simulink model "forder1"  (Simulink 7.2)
settings: Solver=ode45  StartTime=0.0  StopTime=10.0  RelTol=1e-3
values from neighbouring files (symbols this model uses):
  k = 1    [second_init.m]
  ki = 1    [second_init.m]
  tau = 1    [second_init.m]
libraries: simulink x1

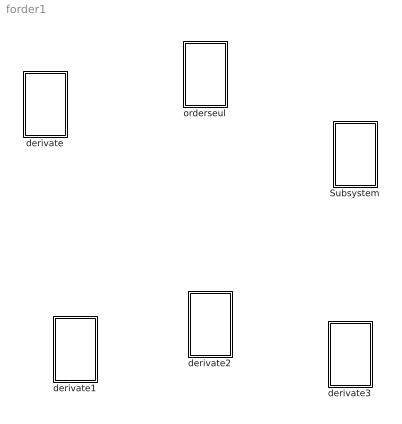
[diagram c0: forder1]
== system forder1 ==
  Subsystem : Subsystem
  derivate : Subsystem
  derivate1 : Subsystem
  derivate2 : Subsystem
  derivate3 : Subsystem
  orderseul : Subsystem

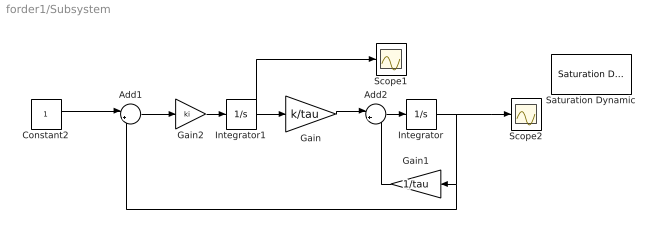
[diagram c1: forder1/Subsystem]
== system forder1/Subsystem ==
  Add1 : Sum  Inputs=|+-  OutDataType=sfix(16)  OutScaling=2^-10
  Add2 : Sum  Inputs=|+-  OutDataType=sfix(16)  OutScaling=2^-10
  Constant2 : Constant  OutDataType=sfix(16)  OutScaling=2^0
  Gain : Gain  Gain=k/tau  ParameterDataType=sfix(16)  ParameterScaling=2^0  OutDataType=sfix(16)  OutScaling=2^0
  Gain1 : Gain  Orientation=left  Gain=1/tau  ParameterDataType=sfix(16)  ParameterScaling=2^0  OutDataType=sfix(16)  OutScaling=2^0
  Gain2 : Gain  Gain=ki  ParameterDataType=sfix(16)  ParameterScaling=2^0  OutDataType=sfix(16)  OutScaling=2^0
  Integrator : Integrator
  Integrator1 : Integrator
  Saturation Dynamic : simulink/Discontinuities/Saturation Dynamic  SystemSampleTime=-1  OutMin=[]  OutMax=[]  OutDataTypeStr=Inherit: Same as second input  OutDataType=sfix(16)  OutScaling=2^-10  DoSatur=off
  Scope1 : Scope
  Scope2 : Scope
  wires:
  Constant2/1 -> Add1/1
  Integrator/1 -> Scope2/1, Gain1/1, Add1/2
  Gain1/1 -> Add2/2
  Gain/1 -> Add2/1
  Add2/1 -> Integrator/1
  Integrator1/1 -> Gain/1, Scope1/1
  Gain2/1 -> Integrator1/1
  Add1/1 -> Gain2/1

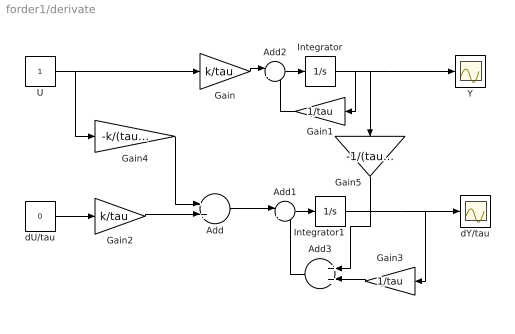
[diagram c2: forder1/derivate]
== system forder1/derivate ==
  Add : Sum  OutDataType=sfix(16)  OutScaling=2^-10
  Add1 : Sum  Inputs=|+-  OutDataType=sfix(16)  OutScaling=2^-10
  Add2 : Sum  Inputs=|+-  OutDataType=sfix(16)  OutScaling=2^-10
  Add3 : Sum  Orientation=left  OutDataType=sfix(16)  OutScaling=2^-10
  Gain : Gain  Gain=k/tau  ParameterDataType=sfix(16)  ParameterScaling=2^0  OutDataType=sfix(16)  OutScaling=2^0
  Gain1 : Gain  Orientation=left  Gain=1/tau  ParameterDataType=sfix(16)  ParameterScaling=2^0  OutDataType=sfix(16)  OutScaling=2^0
  Gain2 : Gain  Gain=k/tau  ParameterDataType=sfix(16)  ParameterScaling=2^0  OutDataType=sfix(16)  OutScaling=2^0
  Gain3 : Gain  Orientation=left  Gain=1/tau  ParameterDataType=sfix(16)  ParameterScaling=2^0  OutDataType=sfix(16)  OutScaling=2^0
  Gain4 : Gain  Gain=-k/(tau^2)  ParameterDataType=sfix(16)  ParameterScaling=2^0  OutDataType=sfix(16)  OutScaling=2^0
  Gain5 : Gain  Orientation=down  Gain=-1/(tau^2)  ParameterDataType=sfix(16)  ParameterScaling=2^0  OutDataType=sfix(16)  OutScaling=2^0
  Integrator : Integrator
  Integrator1 : Integrator
  U : Constant  OutDataType=sfix(16)  OutScaling=2^0
  Y : Scope
  dU/tau : Constant  Value=0  OutDataType=sfix(16)  OutScaling=2^0
  dY/tau : Scope
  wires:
  Integrator/1 -> Y/1, Gain1/1, Gain5/1
  Gain1/1 -> Add2/2
  Gain/1 -> Add2/1
  Add2/1 -> Integrator/1
  U/1 -> Gain/1, Gain4/1
  Integrator1/1 -> dY/tau/1, Gain3/1
  Add1/1 -> Integrator1/1
  dU/tau/1 -> Gain2/1
  Gain2/1 -> Add/2
  Gain4/1 -> Add/1
  Gain3/1 -> Add3/2
  Gain5/1 -> Add3/1
  Add3/1 -> Add1/2
  Add/1 -> Add1/1

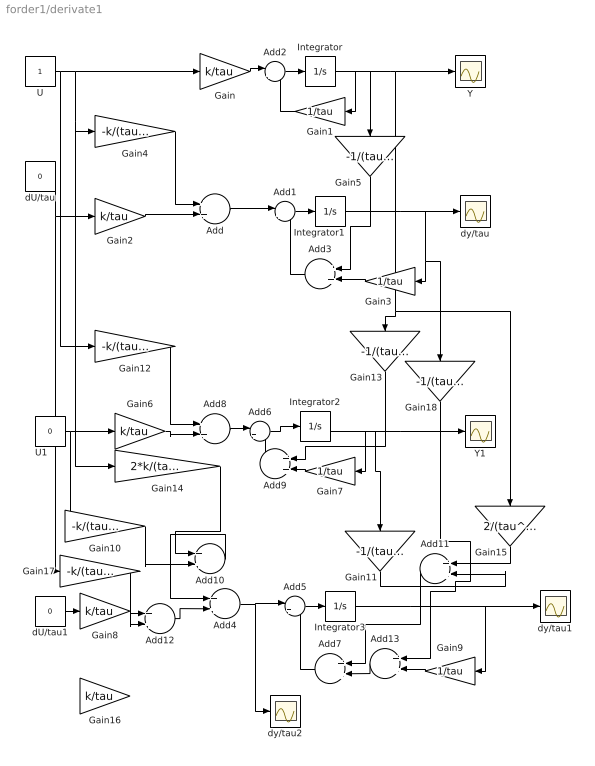
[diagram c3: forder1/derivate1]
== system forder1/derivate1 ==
  Add{,4,8,10,12} (5 alike) : Sum  OutDataType=sfix(16)  OutScaling=2^-10
  Add{1..2,5..6} (4 alike) : Sum  Inputs=|+-  OutDataType=sfix(16)  OutScaling=2^-10
  Add{3,7,9,11,13} (5 alike) : Sum  Orientation=left  OutDataType=sfix(16)  OutScaling=2^-10
  Gain{,2,6,8,16} (5 alike) : Gain  Gain=k/tau  ParameterDataType=sfix(16)  ParameterScaling=2^0  OutDataType=sfix(16)  OutScaling=2^0
  Gain{1,3,7,9} (4 alike) : Gain  Orientation=left  Gain=1/tau  ParameterDataType=sfix(16)  ParameterScaling=2^0  OutDataType=sfix(16)  OutScaling=2^0
  Gain{4,10,12,17} (4 alike) : Gain  Gain=-k/(tau^2)  ParameterDataType=sfix(16)  ParameterScaling=2^0  OutDataType=sfix(16)  OutScaling=2^0
  Gain{5,11,13,18} (4 alike) : Gain  Orientation=down  Gain=-1/(tau^2)  ParameterDataType=sfix(16)  ParameterScaling=2^0  OutDataType=sfix(16)  OutScaling=2^0
  Gain14 : Gain  Gain=2*k/(tau^3)  ParameterDataType=sfix(16)  ParameterScaling=2^0  OutDataType=sfix(16)  OutScaling=2^0
  Gain15 : Gain  Orientation=down  Gain=2/(tau^3)  ParameterDataType=sfix(16)  ParameterScaling=2^0  OutDataType=sfix(16)  OutScaling=2^0
  Integrator{,1..3} (4 alike) : Integrator
  U : Constant  OutDataType=sfix(16)  OutScaling=2^0
  U1 : Constant  Value=0  OutDataType=sfix(16)  OutScaling=2^0
  Y : Scope
  Y1 : Scope
  dU/tau : Constant  Value=0  OutDataType=sfix(16)  OutScaling=2^0
  dU/tau1 : Constant  Value=0  OutDataType=sfix(16)  OutScaling=2^0
  dy/tau : Scope
  dy/tau1 : Scope
  dy/tau2 : Scope
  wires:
  Integrator/1 -> Gain1/1, Gain5/1, Y/1, Gain13/1, Gain15/1
  Gain1/1 -> Add2/2
  Gain/1 -> Add2/1
  Add2/1 -> Integrator/1
  U/1 -> Gain/1, Gain4/1, Gain14/1, Gain12/1
  Integrator1/1 -> dy/tau/1, Gain3/1, Gain18/1
  Add1/1 -> Integrator1/1
  dU/tau/1 -> Gain2/1, Gain17/1
  Gain2/1 -> Add/2
  Gain4/1 -> Add/1
  Gain3/1 -> Add3/2
  Gain5/1 -> Add3/1
  Add3/1 -> Add1/2
  Add/1 -> Add1/1
  Integrator2/1 -> Y1/1, Gain7/1, Gain11/1
  Gain6/1 -> Add8/2
  Add6/1 -> Integrator2/1
  U1/1 -> Gain10/1, Gain6/1
  Integrator3/1 -> dy/tau1/1, Gain9/1
  Add5/1 -> Integrator3/1
  dU/tau1/1 -> Gain8/1
  Add7/1 -> Add5/2
  Add4/1 -> Add5/1, dy/tau2/1
  Gain12/1 -> Add8/1
  Add8/1 -> Add6/1
  Gain7/1 -> Add9/2
  Add9/1 -> Add6/2
  Gain13/1 -> Add9/1
  Gain10/1 -> Add10/2
  Gain14/1 -> Add10/1
  Add10/1 -> Add4/1
  Gain11/1 -> Add11/2
  Gain15/1 -> Add11/1
  Add11/1 -> Add7/1
  Gain8/1 -> Add12/2
  Gain17/1 -> Add12/1
  Add12/1 -> Add4/2
  Gain9/1 -> Add13/2
  Add13/1 -> Add7/2
  Gain18/1 -> Add13/1

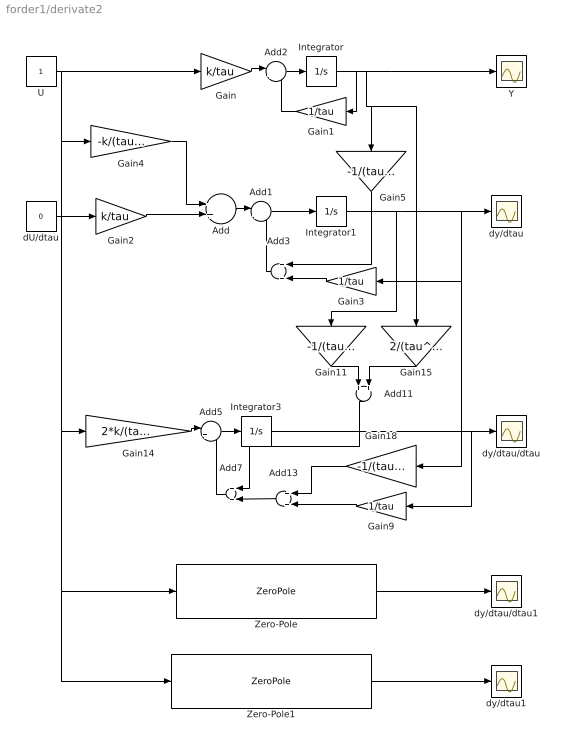
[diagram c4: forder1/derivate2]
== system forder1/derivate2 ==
  Add : Sum  OutDataType=sfix(16)  OutScaling=2^-10
  Add1 : Sum  Inputs=|+-  OutDataType=sfix(16)  OutScaling=2^-10
  Add11 : Sum  Orientation=down  OutDataType=sfix(16)  OutScaling=2^-10
  Add13 : Sum  Orientation=left  OutDataType=sfix(16)  OutScaling=2^-10
  Add2 : Sum  Inputs=|+-  OutDataType=sfix(16)  OutScaling=2^-10
  Add3 : Sum  Orientation=left  OutDataType=sfix(16)  OutScaling=2^-10
  Add5 : Sum  Inputs=|+-  OutDataType=sfix(16)  OutScaling=2^-10
  Add7 : Sum  Orientation=left  OutDataType=sfix(16)  OutScaling=2^-10
  Gain : Gain  Gain=k/tau  ParameterDataType=sfix(16)  ParameterScaling=2^0  OutDataType=sfix(16)  OutScaling=2^0
  Gain1 : Gain  Orientation=left  Gain=1/tau  ParameterDataType=sfix(16)  ParameterScaling=2^0  OutDataType=sfix(16)  OutScaling=2^0
  Gain11 : Gain  Orientation=down  Gain=-1/(tau^2)  ParameterDataType=sfix(16)  ParameterScaling=2^0  OutDataType=sfix(16)  OutScaling=2^0
  Gain14 : Gain  Gain=2*k/(tau^3)  ParameterDataType=sfix(16)  ParameterScaling=2^0  OutDataType=sfix(16)  OutScaling=2^0
  Gain15 : Gain  Orientation=down  Gain=2/(tau^3)  ParameterDataType=sfix(16)  ParameterScaling=2^0  OutDataType=sfix(16)  OutScaling=2^0
  Gain18 : Gain  Orientation=left  Gain=-1/(tau^2)  ParameterDataType=sfix(16)  ParameterScaling=2^0  OutDataType=sfix(16)  OutScaling=2^0
  Gain2 : Gain  Gain=k/tau  ParameterDataType=sfix(16)  ParameterScaling=2^0  OutDataType=sfix(16)  OutScaling=2^0
  Gain3 : Gain  Orientation=left  Gain=1/tau  ParameterDataType=sfix(16)  ParameterScaling=2^0  OutDataType=sfix(16)  OutScaling=2^0
  Gain4 : Gain  Gain=-k/(tau^2)  ParameterDataType=sfix(16)  ParameterScaling=2^0  OutDataType=sfix(16)  OutScaling=2^0
  Gain5 : Gain  Orientation=down  Gain=-1/(tau^2)  ParameterDataType=sfix(16)  ParameterScaling=2^0  OutDataType=sfix(16)  OutScaling=2^0
  Gain9 : Gain  Orientation=left  Gain=1/tau  ParameterDataType=sfix(16)  ParameterScaling=2^0  OutDataType=sfix(16)  OutScaling=2^0
  Integrator : Integrator
  Integrator1 : Integrator
  Integrator3 : Integrator
  U : Constant  OutDataType=sfix(16)  OutScaling=2^0
  Y : Scope
  Zero-Pole : ZeroPole  Zeros=[0 0]  Poles=[-1/tau -1/tau -1/tau]  Gain=[2*k/tau/tau/tau]
  Zero-Pole1 : ZeroPole  Zeros=[0]  Poles=[-1/tau -1/tau ]  Gain=[-k/tau/tau]
  dU/dtau : Constant  Value=0  OutDataType=sfix(16)  OutScaling=2^0
  dy/dtau : Scope
  dy/dtau/dtau : Scope
  dy/dtau/dtau1 : Scope
  dy/dtau1 : Scope
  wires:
  Integrator/1 -> Gain1/1, Gain5/1, Gain15/1, Y/1
  Gain1/1 -> Add2/2
  Gain/1 -> Add2/1
  Add2/1 -> Integrator/1
  U/1 -> Gain/1, Gain4/1, Gain14/1, Zero-Pole/1, Zero-Pole1/1
  Integrator1/1 -> Gain3/1, Gain18/1, dy/dtau/1, Gain11/1
  Add1/1 -> Integrator1/1
  dU/dtau/1 -> Gain2/1
  Gain2/1 -> Add/2
  Gain4/1 -> Add/1
  Gain3/1 -> Add3/2
  Gain5/1 -> Add3/1
  Add3/1 -> Add1/2
  Add/1 -> Add1/1
  Integrator3/1 -> dy/dtau/dtau/1, Gain9/1
  Add5/1 -> Integrator3/1
  Add7/1 -> Add5/2
  Gain14/1 -> Add5/1
  Add11/1 -> Add7/1
  Gain9/1 -> Add13/2
  Add13/1 -> Add7/2
  Gain15/1 -> Add11/2
  Gain11/1 -> Add11/1
  Gain18/1 -> Add13/1
  Zero-Pole/1 -> dy/dtau/dtau1/1
  Zero-Pole1/1 -> dy/dtau1/1

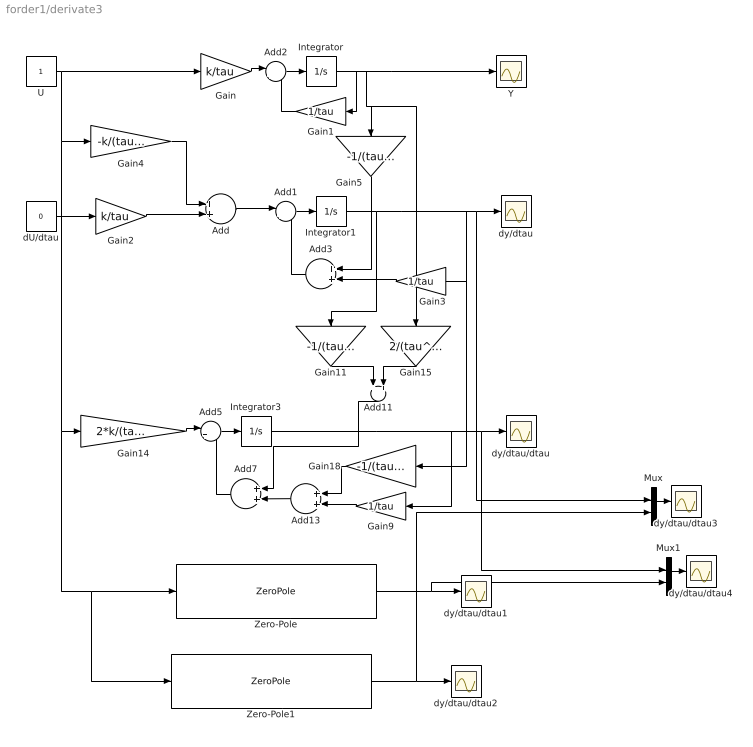
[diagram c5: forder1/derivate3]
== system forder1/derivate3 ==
  Add : Sum  OutDataType=sfix(16)  OutScaling=2^-10
  Add1 : Sum  Inputs=|+-  OutDataType=sfix(16)  OutScaling=2^-10
  Add11 : Sum  Orientation=down  OutDataType=sfix(16)  OutScaling=2^-10
  Add13 : Sum  Orientation=left  OutDataType=sfix(16)  OutScaling=2^-10
  Add2 : Sum  Inputs=|+-  OutDataType=sfix(16)  OutScaling=2^-10
  Add3 : Sum  Orientation=left  OutDataType=sfix(16)  OutScaling=2^-10
  Add5 : Sum  Inputs=|+-  OutDataType=sfix(16)  OutScaling=2^-10
  Add7 : Sum  Orientation=left  OutDataType=sfix(16)  OutScaling=2^-10
  Gain : Gain  Gain=k/tau  ParameterDataType=sfix(16)  ParameterScaling=2^0  OutDataType=sfix(16)  OutScaling=2^0
  Gain1 : Gain  Orientation=left  Gain=1/tau  ParameterDataType=sfix(16)  ParameterScaling=2^0  OutDataType=sfix(16)  OutScaling=2^0
  Gain11 : Gain  Orientation=down  Gain=-1/(tau^2)  ParameterDataType=sfix(16)  ParameterScaling=2^0  OutDataType=sfix(16)  OutScaling=2^0
  Gain14 : Gain  Gain=2*k/(tau^3)  ParameterDataType=sfix(16)  ParameterScaling=2^0  OutDataType=sfix(16)  OutScaling=2^0
  Gain15 : Gain  Orientation=down  Gain=2/(tau^3)  ParameterDataType=sfix(16)  ParameterScaling=2^0  OutDataType=sfix(16)  OutScaling=2^0
  Gain18 : Gain  Orientation=left  Gain=-1/(tau^2)  ParameterDataType=sfix(16)  ParameterScaling=2^0  OutDataType=sfix(16)  OutScaling=2^0
  Gain2 : Gain  Gain=k/tau  ParameterDataType=sfix(16)  ParameterScaling=2^0  OutDataType=sfix(16)  OutScaling=2^0
  Gain3 : Gain  Orientation=left  Gain=1/tau  ParameterDataType=sfix(16)  ParameterScaling=2^0  OutDataType=sfix(16)  OutScaling=2^0
  Gain4 : Gain  Gain=-k/(tau^2)  ParameterDataType=sfix(16)  ParameterScaling=2^0  OutDataType=sfix(16)  OutScaling=2^0
  Gain5 : Gain  Orientation=down  Gain=-1/(tau^2)  ParameterDataType=sfix(16)  ParameterScaling=2^0  OutDataType=sfix(16)  OutScaling=2^0
  Gain9 : Gain  Orientation=left  Gain=1/tau  ParameterDataType=sfix(16)  ParameterScaling=2^0  OutDataType=sfix(16)  OutScaling=2^0
  Integrator : Integrator
  Integrator1 : Integrator
  Integrator3 : Integrator
  Mux : Mux  Inputs=2
  Mux1 : Mux  Inputs=2
  U : Constant  OutDataType=sfix(16)  OutScaling=2^0
  Y : Scope
  Zero-Pole : ZeroPole  Zeros=[0 0]  Poles=[-1/tau -1/tau -1/tau]  Gain=[2*k/tau/tau/tau]
  Zero-Pole1 : ZeroPole  Zeros=[0]  Poles=[-1/tau -1/tau ]  Gain=[-k/tau/tau]
  dU/dtau : Constant  Value=0  OutDataType=sfix(16)  OutScaling=2^0
  dy/dtau : Scope
  dy/dtau/dtau{,1..4} (5 alike) : Scope
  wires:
  Integrator/1 -> Gain1/1, Gain5/1, Gain15/1, Y/1
  Gain1/1 -> Add2/2
  Gain/1 -> Add2/1
  Add2/1 -> Integrator/1
  U/1 -> Gain/1, Gain4/1, Gain14/1, Zero-Pole/1, Zero-Pole1/1
  Integrator1/1 -> Gain3/1, Gain18/1, dy/dtau/1, Mux/1, Gain11/1
  Add1/1 -> Integrator1/1
  dU/dtau/1 -> Gain2/1
  Gain2/1 -> Add/2
  Gain4/1 -> Add/1
  Gain3/1 -> Add3/2
  Gain5/1 -> Add3/1
  Add3/1 -> Add1/2
  Add/1 -> Add1/1
  Integrator3/1 -> Gain9/1, dy/dtau/dtau/1, Mux1/1
  Add5/1 -> Integrator3/1
  Add7/1 -> Add5/2
  Gain14/1 -> Add5/1
  Add11/1 -> Add7/1
  Gain9/1 -> Add13/2
  Add13/1 -> Add7/2
  Gain15/1 -> Add11/2
  Gain11/1 -> Add11/1
  Gain18/1 -> Add13/1
  Zero-Pole/1 -> dy/dtau/dtau1/1, Mux1/2
  Zero-Pole1/1 -> dy/dtau/dtau2/1, Mux/2
  Mux/1 -> dy/dtau/dtau3/1
  Mux1/1 -> dy/dtau/dtau4/1

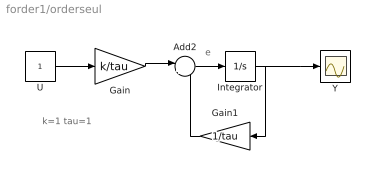
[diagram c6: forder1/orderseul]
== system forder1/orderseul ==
  note: e
  note: k=1 tau=1
  Add2 : Sum  Inputs=|+-  OutDataType=sfix(16)  OutScaling=2^-10
  Gain : Gain  Gain=k/tau  ParameterDataType=sfix(16)  ParameterScaling=2^0  OutDataType=sfix(16)  OutScaling=2^0
  Gain1 : Gain  Orientation=left  Gain=1/tau  ParameterDataType=sfix(16)  ParameterScaling=2^0  OutDataType=sfix(16)  OutScaling=2^0
  Integrator : Integrator
  U : Constant  OutDataType=sfix(16)  OutScaling=2^0
  Y : Scope
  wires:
  Integrator/1 -> Y/1, Gain1/1
  Gain1/1 -> Add2/2
  Gain/1 -> Add2/1
  Add2/1 -> Integrator/1
  U/1 -> Gain/1
